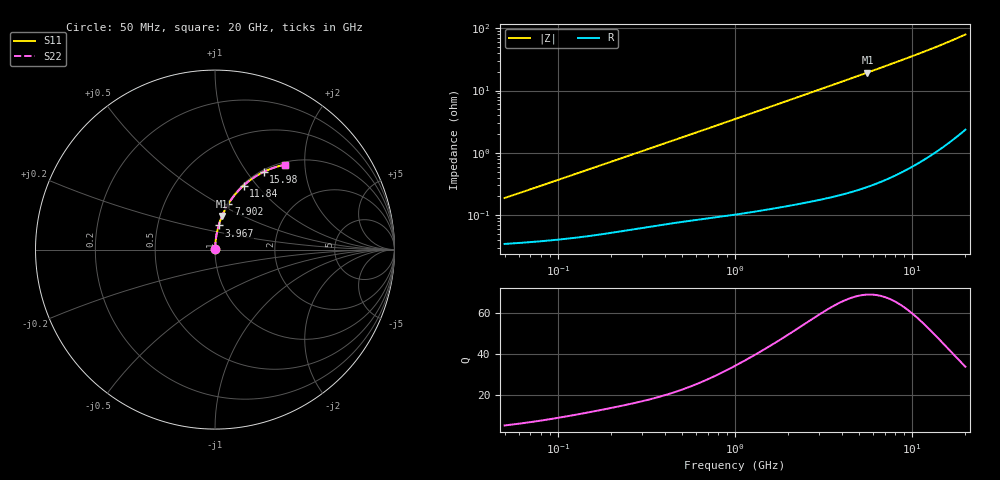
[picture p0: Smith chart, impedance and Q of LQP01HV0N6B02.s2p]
!Murata Part Number: LQP01HV0N6B02
!These Parameters are Measured in Series Mode Connection
!  o--[Z]--o
!Port1  Port2
!  o-------o
!Freq. Start=50[MHz] Stop=20[GHz], 401[Steps]
# Hz S RI R 50
!Freq.(Hz) S11(Real) S11(Imag) S21(Real) S21(Imag) S12(Real) S12(Imag) S22(Real) S22(Imag)
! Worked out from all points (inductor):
!   401 points, 50 MHz to 20 GHz, reference 50 ohm
!   read as one part in series: L = 586 pH near 51.52 MHz
!   highest Q = 68.7 at 5.599 GHz (marker M1), where L = 554 pH
!   S11 on the Smith chart (normalised r, x): 50 MHz: 1.00, +0.00; 3.967 GHz: 1.00, +0.28; 7.902 GHz: 1.01, +0.56; 11.84 GHz: 1.02, +0.86; 15.98 GHz: 1.03, +1.20; 20 GHz: 1.05, +1.59
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5e7  0.000348 0.00185  0.9997 -0.00185  0.9997 -0.00185  0.000348 0.00185
5.152053e7  0.00035 0.00191  0.9996 -0.00191  0.9996 -0.00191  0.00035 0.00191
5.552724e7  0.000356 0.00205  0.9996 -0.00205  0.9996 -0.00205  0.000356 0.00205
1.364002e8  0.00047 0.00494  0.9995 -0.00494  0.9995 -0.00494  0.00047 0.00494
3.721004e8  0.00086 0.0132  0.9991 -0.0132  0.9991 -0.0132  0.00086 0.0132
6.380365e8  0.00135 0.0223  0.9986 -0.0223  0.9986 -0.0223  0.00135 0.0223
1e9  0.00223 0.0347  0.9978 -0.0347  0.9978 -0.0347  0.00223 0.0347
1.714689e9  0.00481 0.0591  0.9952 -0.0591  0.9952 -0.0591  0.00481 0.0591
2.728004e9  0.0105 0.0933  0.9895 -0.0933  0.9895 -0.0933  0.0105 0.0933
3.967106e9  0.0206 0.1344  0.9794 -0.1344  0.9794 -0.1344  0.0206 0.1344
4.748272e9  0.0287 0.1598  0.9713 -0.1598  0.9713 -0.1598  0.0287 0.1598
5.598765e9  0.0391 0.1868  0.9609 -0.1868  0.9609 -0.1868  0.0391 0.1868
7.442007e9  0.067 0.2426  0.933 -0.2426  0.933 -0.2426  0.067 0.2426
7.901521e9  0.075 0.2559  0.925 -0.2559  0.925 -0.2559  0.075 0.2559
9.745021e9  0.1112 0.3062  0.8888 -0.3062  0.8888 -0.3062  0.1112 0.3062
1.082228e10  0.1351 0.3332  0.8649 -0.3332  0.8649 -0.3332  0.1351 0.3332
1.183995e10  0.1593 0.3568  0.8407 -0.3568  0.8407 -0.3568  0.1593 0.3568
1.375312e10  0.2086 0.3961  0.7914 -0.3961  0.7914 -0.3961  0.2086 0.3961
1.597544e10  0.2707 0.4328  0.7293 -0.4328  0.7293 -0.4328  0.2707 0.4328
1.828096e10  0.3391 0.4602  0.6609 -0.4602  0.6609 -0.4602  0.3391 0.4602
1.940974e10  0.3733 0.4696  0.6267 -0.4696  0.6267 -0.4696  0.3733 0.4696
2e10  0.3914 0.4735  0.6086 -0.4735  0.6086 -0.4735  0.3914 0.4735
